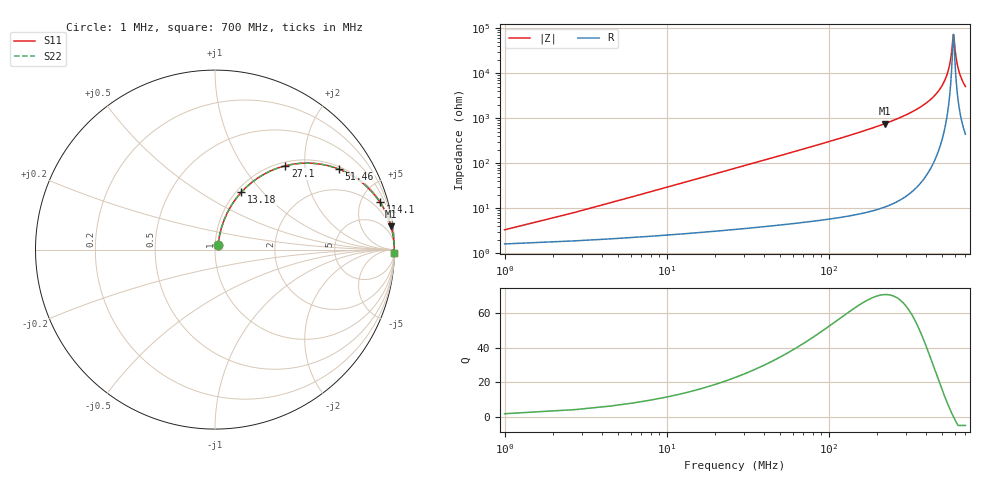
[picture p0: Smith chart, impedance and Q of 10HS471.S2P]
! Coilcraft 1008HS-471 Chip Inductor
! 02 July 2002
# MHZ S MA R 50
!Freq  MagS11  AngS11  MagS21  AngS21  MagS12  AngS12  MagS22  AngS22
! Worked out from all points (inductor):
!   403 points, 1 MHz to 700 MHz, reference 50 ohm
!   read as one part in series: L = 465 nH near 4.48 MHz
!   highest Q = 70.8 at 222 MHz (marker M1), where L = 541 nH
!   self-resonance near 590.9 MHz
!   S11 on the Smith chart (normalised r, x): 1 MHz: 1.03, +0.06; 13.18 MHz: 1.06, +0.77; 27.1 MHz: 1.07, +1.59; 51.46 MHz: 1.09, +3.03; 114.1 MHz: 1.12, +6.93; 700 MHz: open
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1  0.03289 59.2  0.9836 -1.6  0.9836 -1.6  0.03289 59.2
6.22  0.1763 72.8  0.9628 -10.1  0.9628 -10.1  0.1763 72.8
9.7  0.2675 69.4  0.9401 -15.5  0.9401 -15.5  0.2675 69.4
13.18  0.352 65.4  0.9113 -20.6  0.9113 -20.6  0.352 65.4
27.1  0.6092 50.0  0.7671 -37.5  0.7671 -37.5  0.6092 50.0
51.46  0.824 32.9  0.5437 -55.5  0.5437 -55.5  0.824 32.9
77.56  0.9101 23.2  0.3946 -65.5  0.3946 -65.5  0.9101 23.2
114.1  0.9562 16.0  0.2761 -73.0  0.2761 -73.0  0.9562 16.0
117.58  0.9587 15.5  0.268 -73.5  0.268 -73.5  0.9587 15.5
221.98  0.9895 7.5  0.131 -81.7  0.131 -81.7  0.9895 7.5
234.16  0.9908 7.0  0.1221 -82.2  0.1221 -82.2  0.9908 7.0
350.74  0.9968 3.6  0.06301 -85.3  0.06301 -85.3  0.9968 3.6
467.32  0.9985 1.6  0.02742 -86.0  0.02742 -86.0  0.9985 1.6
512.56  0.9986 0.9  0.01657 -84.8  0.01657 -84.8  0.9986 0.9
545.62  0.9987 0.5  0.009337 -81.6  0.009337 -81.6  0.9987 0.5
568.24  0.9987 0.3  0.004734 -73.4  0.004734 -73.4  0.9987 0.3
583.9  0.9986 0.1  0.001957 -45.6  0.001957 -45.6  0.9986 0.1
589.12  0.9986 0.0  0.00143 -15.0  0.00143 -15.0  0.9986 0.0
592.6  0.9986 -0.0  0.001425 12.6  0.001425 12.6  0.9986 -0.0
613.48  0.9985 -0.2  0.004552 71.2  0.004552 71.2  0.9985 -0.2
637.84  0.9984 -0.5  0.008953 79.7  0.008953 79.7  0.9984 -0.5
700  0.9981 -1.1  0.01972 83.8  0.01972 83.8  0.9981 -1.1
